PROGRAM PRG_READ_List
VAR
	fbUA_ConnectEx			: UA_Connect;
	SessionConnectInfoEx	: ST_UASessionConnectInfo;
	sOpcUA_URL				: STRING(MAX_STRING_LENGTH);
	nConnectionHdl			: DWORD;

	fbUA_GetNamespaceIndex 	: UA_GetNamespaceIndex;
	nNamespaceIndex			: UINT;
	fbUA_NodeGetHandleList	: UA_NodeGetHandleList;
	
	NodeIDs					: ARRAY [1..nMaxNodeIDsInList] OF ST_UANodeID;
	nNodeHdls				: ARRAY [1..nMaxNodeIDsInList] OF DWORD;

	fbUA_ReadList			: UA_ReadList;
	NodeIDCount				: UINT := 2;
	NodeHdlCount			: UINT := 2; 
	stIndexRange			: ARRAY [1..nMaxIndexRange] OF ST_UAIndexRange;
	nIndexRangeCount		: UINT;
	stNodeAddInfo			: ARRAY [1..nMaxNodeIDsInList] OF ST_UANodeAdditionalInfo;
	stReadListData			: ST_ReadListData; // memory block must contain the Data[], NodeErrorIDs[], TimeStamps[] and cbData_R[]
	cbData					: ARRAY [1..nMaxNodeIDsInList] OF UDINT; (* Bytes to be actually Read *)
	cbData_R				: UDINT;
	cbDataTotal				: UDINT; 
	
	fbUA_NodeReleaseHandleList	: UA_NodeReleaseHandleList;

	fbUA_Disconnect		: UA_Disconnect;

	iState		: INT;
	bTest		: BOOL:= TRUE;
	bDone		: BOOL;
	bBusy		: BOOL;
	bError		: BOOL;
	nErrorID	: DWORD;
END_VAR


CASE iState OF
0:	(* idle *)
	IF bTest THEN
		bTest		:= FALSE;
		bError		:= FALSE;
		nErrorID	:= 0;

		SessionConnectInfoEx.tConnectTimeout 		:= T#1M;
		SessionConnectInfoEx.tSessionTimeout 		:= T#1M;
		SessionConnectInfoEx.sApplicationName		:= '';
		SessionConnectInfoEx.eSecurityMode 			:= eUASecurityMsgMode_None;
		SessionConnectInfoEx.eSecurityPolicyUri 	:= eUASecurityPolicy_None;
		SessionConnectInfoEx.eTransportProfileUri 	:= eUATransportProfileUri_UATcp;

		iState	:= iState + 1;
	END_IF

1:	(* open UA session *)
	fbUA_ConnectEx(
		Execute				:= TRUE,
		ServerURL			:= sOpcUaServerUrl,
		SessionConnectInfo  := SessionConnectInfoEx,
		Timeout				:= T#2M,
		ConnectionHdl		=> nConnectionHdl
	);

	IF NOT fbUA_ConnectEx.Busy THEN
		fbUA_ConnectEx(Execute := FALSE);

		IF NOT fbUA_ConnectEx.Error THEN
			(* session open *)
			iState := iState + 1;
		ELSE
			bError			:= TRUE;
			nErrorID		:= fbUA_ConnectEx.ErrorID;
			nConnectionHdl	:= 0;
			iState 			:= 0; (* idle *)
		END_IF
	END_IF


2:	(* GetNS Index *)
	fbUA_GetNamespaceIndex(
		Execute			:= TRUE,
		ConnectionHdl	:= nConnectionHdl,
		NamespaceUri	:= sNamespaceUri,
		NamespaceIndex	=> nNamespaceIndex
	);

	IF NOT fbUA_GetNamespaceIndex.Busy THEN
		fbUA_GetNamespaceIndex(Execute := FALSE);
		IF NOT fbUA_GetNamespaceIndex.Error THEN
			(* session closed *)
			iState 		:= iState + 1; (* idle *)
		ELSE
			bError		:= TRUE;
			nErrorID	:= fbUA_GetNamespaceIndex.ErrorID;
			iState 		:= 6; (* idle *)
		END_IF
	END_IF


3:	(* Get Node Handle *)
	
	NodeIDs[1].eIdentifierType := eUAIdentifierType_String;
	NodeIDs[1].nNamespaceIndex := nNamespaceIndex;
	NodeIDs[1].sIdentifier	:= 'MAIN.iVar1';
	
	NodeIDs[2].eIdentifierType := eUAIdentifierType_String;
	NodeIDs[2].nNamespaceIndex := nNamespaceIndex;
	NodeIDs[2].sIdentifier	:= 'MAIN.iVar2';

	fbUA_NodeGetHandleList(
		Execute			:= TRUE,
		ConnectionHdl	:= nConnectionHdl,
		NodeIDCount 	:= NodeIDCount,
		NodeIDs			:= NodeIDs,
		NodeHdls		=> nNodeHdls
	);

	IF NOT fbUA_NodeGetHandleList.Busy THEN
		fbUA_NodeGetHandleList(Execute := FALSE);

		IF NOT fbUA_NodeGetHandleList.Error THEN
			(* session closed *)
			iState 		:= iState + 1; (* idle *)
		ELSE
			bError		:= TRUE;
			nErrorID	:= fbUA_NodeGetHandleList.ErrorID;
			iState 		:= 6; (* idle *)
		END_IF
	END_IF

	
4: 	(* UA_Read *)
	cbData[1] := SIZEOF(stReadListData.nIntVar1);
	cbData[2] := SIZEOF(stReadListData.nIntVar2);
	cbDataTotal := SIZEOF(stReadListData);
	fbUA_ReadList(
		Execute			:= TRUE,
		ConnectionHdl	:= nConnectionHdl,
		NodeHdlCount	:= NodeHdlCount, // 2
		NodeHdls		:= nNodeHdls,
		stNodeAddInfo 	:= stNodeAddInfo,
		pVariable		:= ADR(stReadListData),
		cbData			:= cbData ,
		cbDataTotal		:= cbDataTotal		
		);

	IF NOT fbUA_ReadList.Busy THEN
		fbUA_ReadList( Execute := FALSE, cbData_R => cbData_R);

		IF NOT fbUA_ReadList.Error THEN
			(* session closed *)
			iState 		:= iState + 1; (* idle *)
		ELSE
			bError		:= TRUE;
			nErrorID	:= fbUA_ReadList.ErrorID;
			iState 		:= 6; (* idle *)
		END_IF
	END_IF


5:	(* Release Node Handle *)
	fbUA_NodeReleaseHandleList(
		Execute			:= TRUE,
		ConnectionHdl	:= nConnectionHdl,
		NodeHdlCount	:= NodeHdlCount,
		NodeHdls		:= nNodeHdls
	);

	IF NOT fbUA_NodeReleaseHandleList.Busy THEN
		fbUA_NodeReleaseHandleList(Execute := FALSE);

		IF NOT fbUA_NodeReleaseHandleList.Error THEN
			(* session closed *)
			iState 		:= iState + 1; (* idle *)
		ELSE
			bError		:= TRUE;
			nErrorID	:= fbUA_NodeReleaseHandleList.ErrorID;
			iState 		:= 6; (* idle *)
		END_IF
	END_IF


6:	(* close session *)
	fbUA_Disconnect(
		Execute			:= TRUE,
		ConnectionHdl	:= nConnectionHdl
	);

	IF NOT fbUA_Disconnect.Busy THEN
		fbUA_Disconnect(Execute := FALSE);
		bBusy := FALSE;
		IF NOT fbUA_Disconnect.Error THEN
			(* session closed *)
			iState 		:= 0; (* idle *)
			IF NOT bError THEN 
				bDone 	:= TRUE;
			END_IF
		ELSE
			bError			:= TRUE;
			nErrorID		:= fbUA_Disconnect.ErrorID;
			iState 			:= 0; (* idle *)
			nConnectionHdl	:= 0;
		END_IF
	END_IF
END_CASE

END_PROGRAM
